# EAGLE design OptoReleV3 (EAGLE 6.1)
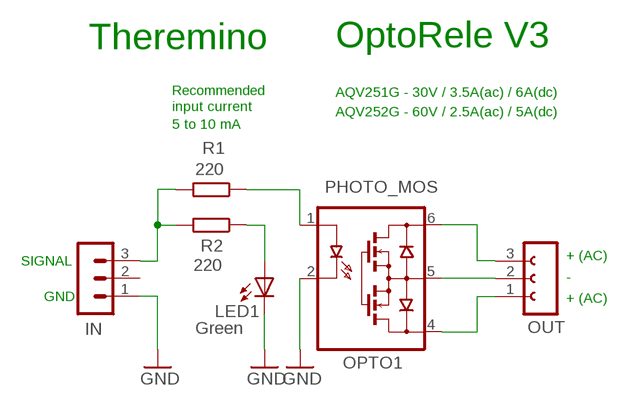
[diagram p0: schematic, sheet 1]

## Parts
IN  MA03-1N  [MA03-1]
LED1  Green  LED3MM_F  [LED3MM]
OPTO1  PHOTO_MOS  [DIL06]
OUT  CN-03"  [CN-03]
R1  220  R-EU_0204/2V  [0204V]
R2  220  R-EU_0204/2V  [0204V]

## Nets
GND: IN.1 LED1.K(C) OPTO1.2
N$1: OPTO1.6 OUT.3
N$2: OPTO1.5 OUT.2
N$3: OPTO1.4 OUT.1
N$4: LED1.A R2.1
N$5: OPTO1.1 R1.1
SIGNAL: IN.3 R1.2 R2.2
Unconnected: IN.2

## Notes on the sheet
- Theremino | OptoRele V3
- Recommended | AQV251G - 30V / 3.5A(ac) / 6A(dc)
- input current
- AQV252G - 60V / 2.5A(ac) / 5A(dc)
- 5 to 10 mA
- + (AC)
- SIGNAL
- -
- GND | + (AC)

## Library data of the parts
IN = 03-con-lstb-M:MA03-1: PIN HEADER
LED1 = 00-LIVIO:LED: LEDS
OPTO1 = 00-LIVIO:PHOTO_MOS: PHOTO MOS
OUT = 01-Connettori_Vite_2.54:CN-03: Screw connector - Green - Spacing 2.54
R1 R2 = 00-LIVIO:R-EU_: RESISTOR, European symbol

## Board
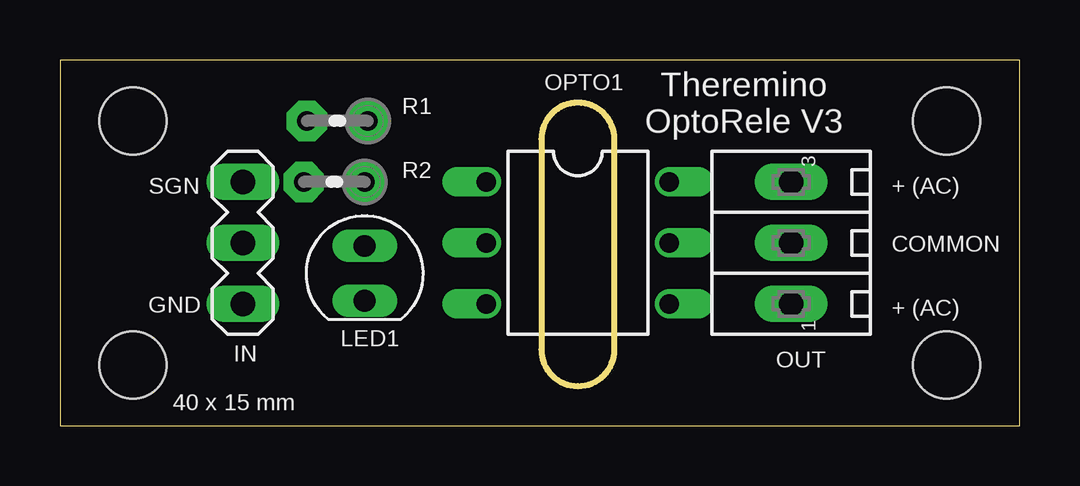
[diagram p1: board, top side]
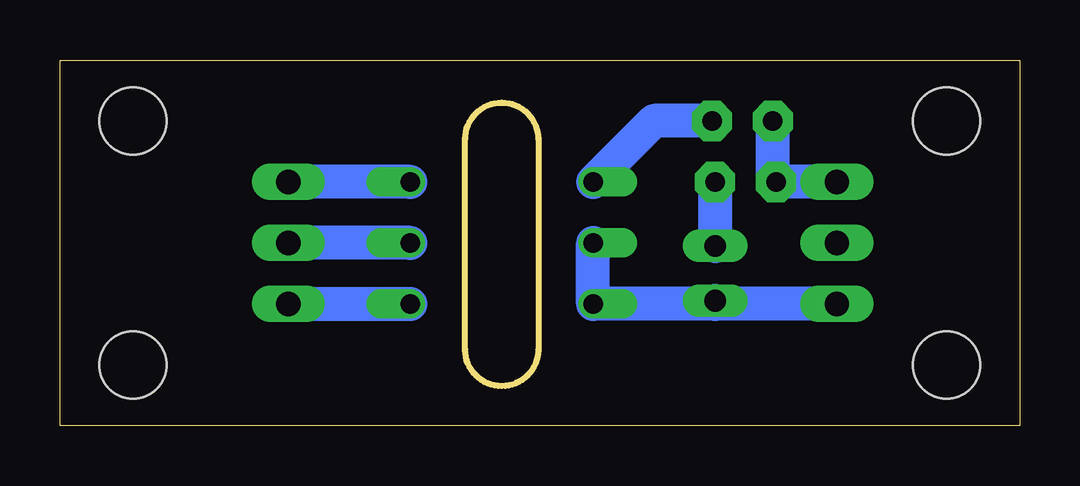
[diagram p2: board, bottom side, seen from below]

Size 40.01 x 15.24 mm. Coordinates in mm from the lower left corner, seen from the top.
Outline: 40.01,15.24 0,15.24 0,0 40.01,0 40.01,15.24
Outline: 20.07,11.94 20.07,3.17 arc180 23.11,3.17 23.11,11.94 arc180 20.07,11.94
Copper layers (1*16): Top 0.035mm / dielectric 1.5mm / Bottom 0.035mm
Design rules: minimum track width 10mil, minimum drill 31mil, track to track 31mil, track to pad 31mil, pad to pad 31mil, via to via 31mil, smd to smd 31mil, copper to edge 31mil, drill to drill 8mil, minimum pad ring 5mil, minimum via ring 8mil, stop-mask expansion 4mil, vias tented up to drill 0mil, thermal gap 47mil
Holes 2.8 mm at 3.05,2.54 3.05,12.7 36.96,2.54 36.96,12.7

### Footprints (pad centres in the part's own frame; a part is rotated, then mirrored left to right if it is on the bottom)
MA03-1 = drill 1.016 long: 1 -2.54,0; 2 0,0; 3 2.54,0
LED3MM = drill 0.9 long: A -1.016,0; K 1.27,0
DIL06 = drill 0.813 offset: 1 -2.54,-3.81; 2 0,-3.81; 3 2.54,-3.81; 4 2.54,3.81; 5 0,3.81; 6 -2.54,3.81
CN-03 = drill 1.016 pad 1.422 long: 1 -2.54,0; 2 0,0; 3 2.54,0
0204V = drill 0.813 pad 1.676 octagon: 1 -1.27,0; 2 1.27,0

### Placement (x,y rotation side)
IN  7.62,7.62 90 top
LED1  12.7,6.48 270 top
OPTO1  21.59,7.62 270 top
OUT  30.48,7.62 90 top
R1  11.56,12.7 180 top
R2  11.43,10.16 180 top

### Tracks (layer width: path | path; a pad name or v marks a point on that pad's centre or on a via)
GND
  Bottom 1.422: IN.1 12.7,5.08 | 12.7,5.08 17.78,5.08 OPTO1.2 | LED1.K 12.7,5.08
N$1
  Bottom 1.422: OPTO1.6 OUT.3
N$2
  Bottom 1.422: OPTO1.5 OUT.2
N$3
  Bottom 1.422: OUT.1 OPTO1.4
N$4
  Bottom 1.422: R2.1 LED1.A
N$5
  Bottom 1.422: R1.1 15.24,12.7 OPTO1.1
SIGNAL
  Bottom 1.422: IN.3 R2.2 10.29,10.16 R1.2

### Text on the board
tNames: Theremino | OptoRele V3 | SGN | + (AC) | COMMON | GND | + (AC) | 40 x 15 mm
